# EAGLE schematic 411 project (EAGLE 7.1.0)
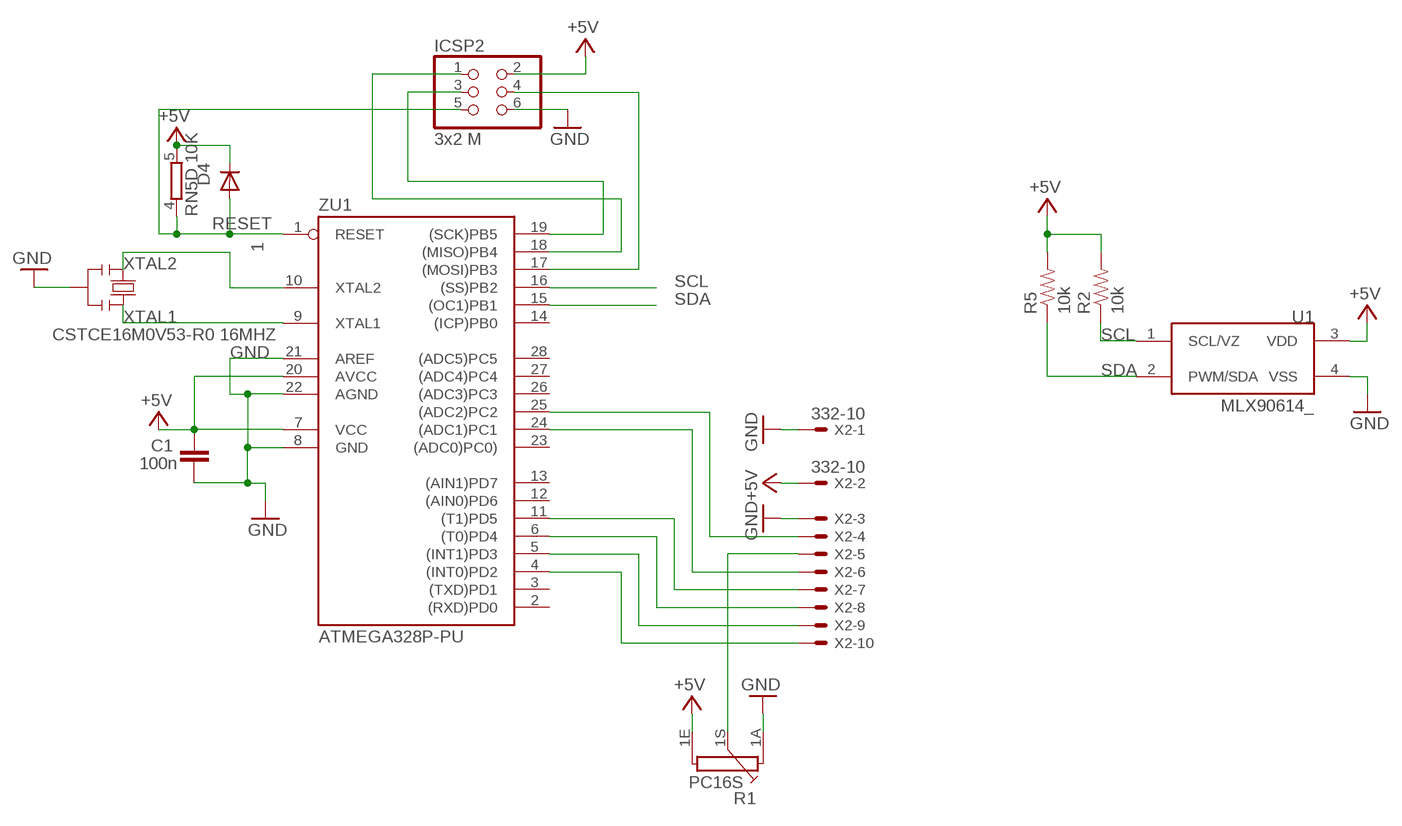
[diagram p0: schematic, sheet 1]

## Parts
C1  100n  C-EU0603-RND  [C0603-ROUND]
D4  1  DIODE-MINIMELF  [MINIMELF]
ICSP2  3x2 M  PINHD-2X3  [2X03]
R1  PC16S  [PC16S]
R2  10k  RESISTOR0402-RES  [0402-RES]
R5  10k  RESISTOR0402-RES  [0402-RES]
RN5  10K  4R-NCAY16  [CAY16]
U1  MLX90614_  [TO-39]
X2  332-10  [332-10]
Y3  CSTCE16M0V53-R0 16MHZ  RESONATORMU  [RESONATOR]
ZU1  ATMEGA328P-PU  [DIL28-3]

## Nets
+5V [usbvcc]: C1.2 D4.C ICSP2.2 R1.1E R2.2 R5.2 RN5.5 U1.3(VDD) X2.2 ZU1.7(VCC) ZU1.20(AVCC)
GND [gnd]: C1.1 ICSP2.6 R1.1A U1.4(VSS) X2.1 X2.3 Y3.2 ZU1.8(GND) ZU1.21(AREF) ZU1.22(AGND)
MISO1: ICSP2.1 ZU1.18((MISO)PB4)
MOSI1: ICSP2.4 ZU1.17((MOSI)PB3)
N$1: X2.10 ZU1.4((INT0)PD2)
N$2: X2.9 ZU1.5((INT1)PD3)
N$3: X2.8 ZU1.6((T0)PD4)
N$4: X2.7 ZU1.11((T1)PD5)
N$5: X2.6 ZU1.24((ADC1)PC1)
N$6: X2.4 ZU1.25((ADC2)PC2)
N$7: R1.1S X2.5
RESET: D4.A ICSP2.5 RN5.4 ZU1.1(RESET)
SCK1: ICSP2.3 ZU1.19((SCK)PB5)
SCL: R2.1 U1.1(SCL/VZ) ZU1.16((SS)PB2)
SDA: R5.1 U1.2(PWM/SDA) ZU1.15((OC1)PB1)
XTAL1: Y3.3 ZU1.9(XTAL1)
XTAL2: Y3.1 ZU1.10(XTAL2)
Unconnected: RN5.1 RN5.2 RN5.3 RN5.6 RN5.7 RN5.8 ZU1.2((RXD)PD0) ZU1.3((TXD)PD1) ZU1.12((AIN0)PD6) ZU1.13((AIN1)PD7) ZU1.14((ICP)PB0) ZU1.23((ADC0)PC0)) ZU1.26((ADC3)PC3) ZU1.27((ADC4)PC4) ZU1.28((ADC5)PC5)

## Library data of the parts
C1 = SmartPrj:C-EU: CAPACITOR, European symbol
D4 = diode:DIODE-: DIODE
ICSP2 = SmartPrj:PINHD-2X3: PIN HEADER
R1 = piher:PC16S: POTENTIOMETER single carbon potentiometer, 16 mm, S3ROH; OC_FARNELL: 4452940; OC_NEWARK: unknown
R2 R5 = SparkFun:RESISTOR: Resistor
RN5 = resistor-dil:4R-N: Array Chip Resistor Source: RS Component / Phycomp
U1 = SparkFun:MLX90614: Melexis IR Thermometer
X2 = con-garry:332-10: 10 Pin - 2mm Dual Row Source: www.mpe-connector.de / garry_shortform_2012.pdf
Y3 = SmartPrj:RESONATOR
ZU1 = SmartPrj:ATMEGA328P-: MICROCONTROLLER 4 Kbytes FLASH 128 bytes SRAM 256 bytes EEPROM UART 6-channel 10 bit ADC

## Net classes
1 power: width 0.61 mm, drill 0.61 mm, clearance 0.254 mm
2 gnd: width 0.305 mm, drill 0.559 mm, clearance 0.254 mm
3 usbvcc: width 0.508 mm, drill 0.61 mm, clearance 0.254 mm
4 aref: width 0.406 mm, drill 0.61 mm, clearance 0.254 mm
